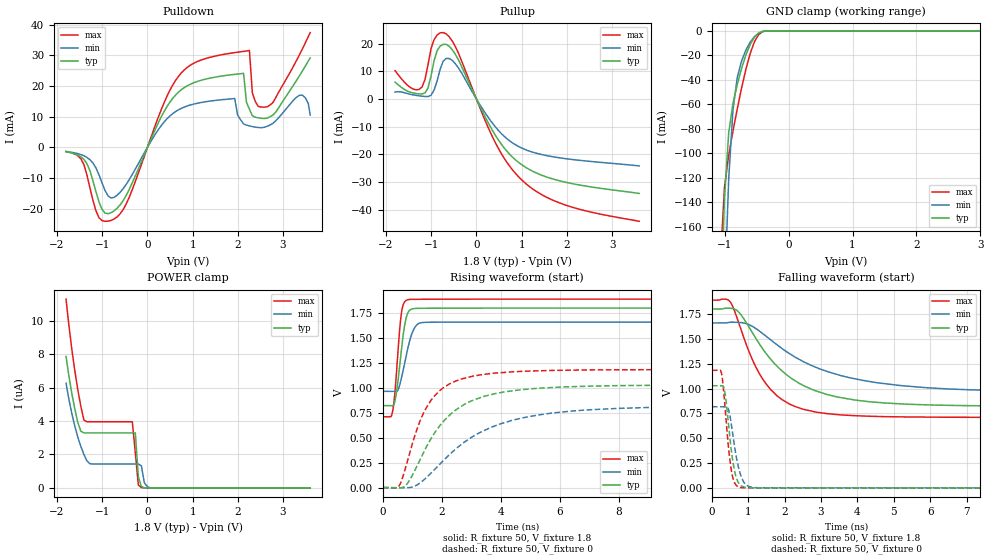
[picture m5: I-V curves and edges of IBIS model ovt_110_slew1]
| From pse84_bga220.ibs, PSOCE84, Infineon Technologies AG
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[Model] ovt_110_slew1
Model_type I/O
Enable   Active-High
Vinl  =  0.54
Vinh  =  1.26
Vmeas =  0.9
Cref  =  15e-12
| Capacitance   typ   min   max
C_comp   1.39974e-12   1.35992e-12   1.44753e-12
| Variables   typ   min   max
[GND Clamp Reference]   0   0   0
[POWER Clamp Reference]   1.8   1.66   1.89
[Pulldown Reference]   0   0   0
[Pullup Reference]   1.8   1.66   1.89
[Temperature Range]   25   125   -40
[Voltage Range]   1.8   1.66   1.89
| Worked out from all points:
|   slope of the pulldown table from 0 to 0.27 V, typ, clamps not added: 30.3 ohm
|   slope of the pullup table from 0 to 0.27 V, typ, clamps not added: 30.5 ohm
|   GND clamp passes 1 mA (typ) near -0.43 V on its own axis
|   falling waveform, R_fixture 50, V_fixture 1.8: 20-80 % time 1.54ns typ, 2.34ns min, 992ps max; typ from 1.8 V to 0.822 V
|   falling waveform, R_fixture 50, V_fixture 0: 20-80 % time 200ps typ, 233ps min, 180ps max; typ from 1.03 V to 0 V
|   rising waveform, R_fixture 50, V_fixture 1.8: 20-80 % time 234ps typ, 323ps min, 184ps max; typ from 0.822 V to 1.8 V
|   rising waveform, R_fixture 50, V_fixture 0: 20-80 % time 1.56ns typ, 2.46ns min, 1.04ns max; typ from 0 V to 1.03 V
[GND Clamp]
| Voltage   I(typ)   I(min)   I(max)
-1.271V   -717.5mA   -832.8mA   -643.6mA
-1.07V    -241.9mA   -348.3mA   -192.2mA
-1.003V   -137.2mA   -218.1mA   -128.1mA
-936.6mV  -83.06mA   -120.7mA   -101.3mA
-869.7mV  -59.26mA   -64.32mA   -81.77mA
-802.8mV  -43.7mA    -38.08mA   -63.69mA
-735.9mV  -30.76mA   -24.63mA   -46.83mA
-602.1mV  -11.27mA   -9.362mA   -18.72mA
-535.2mV  -5.241mA   -4.803mA   -9.042mA
-468.3mV  -1.746mA   -1.965mA   -3.086mA
-334.5mV  -35.9uA    -120.8uA   -33.39uA
3.6V      0A         0A         0A
[POWER Clamp]
| Voltage   I(typ)   I(min)   I(max)
-1.8V     7.872uA    6.273uA    11.31uA
-1.672V   5.671uA    4.461uA    8.32uA
-1.539V   3.91uA     3.037uA    5.87uA
-1.405V   3.295uA    2.008uA    4.063uA
-1.271V   3.295uA    1.447uA    3.964uA
-334.5mV  3.295uA    1.429uA    3.964uA
-267.6mV  3.295uA    1.429uA    2.099uA
-200.7mV  664.1nA    1.429uA    166.6nA
-133.8mV  69.92nA    1.319uA    14.86nA
-66.9mV   7.33nA     291.5nA    4.066nA
62.07mV   0A         0A         0A
3.6V      0A         0A         0A
[Pulldown]
| Voltage   I(typ)   I(min)   I(max)
-1.8V     -1.439mA   -1.35mA    -1.318mA
-1.405V   -3.905mA   -2.719mA   -5.569mA
-1.07V    -17.75mA   -8.962mA   -22.94mA
-735.9mV  -20.66mA   -16.27mA   -23.33mA
806.9mV   19.41mA    13.09mA    25.15mA
1.93V     23.81mA    15.95mA    30.9mA
2.126V    24.14mA    7.657mA    31.3mA
2.256V    12.46mA    7.006mA    31.58mA
2.321V    10.32mA    6.784mA    17.72mA
2.647V    9.522mA    6.888mA    13.22mA
3.364V    23.4mA     17mA       30.24mA
3.6V      29.19mA    10.55mA    37.43mA
[Pullup]
| Voltage   I(typ)   I(min)   I(max)
-1.8V     6.105mA    2.518mA    10.28mA
-1.271V   1.855mA    1.166mA    3.446mA
-1.137V   2.224mA    912.4uA    7.05mA
-1.07V    4.038mA    883.8uA    12.45mA
-936.6mV  13.89mA    3.25mA     21.49mA
-802.8mV  19.14mA    10.79mA    23.94mA
-669mV    19.74mA    14.67mA    23.55mA
-401.4mV  14.31mA    11.31mA    16.73mA
434.5mV   -13.51mA   -10.38mA   -16.28mA
993.1mV   -23.65mA   -17.65mA   -29.11mA
1.89V     -29.77mA   -21.37mA   -37.87mA
3.6V      -34.13mA   -24.18mA   -44.2mA
[Ramp]
dV/dt_r   0.617231/1.56317n  0.490169/2.45731n  0.709901/1.03544n
dV/dt_f   0.586718/1.54262n  0.416735/2.33681n  0.708163/0.991622n
R_load = 50
[Falling Waveform]
R_fixture = 50
V_fixture = 1.8
V_fixture_min = 1.66
V_fixture_max = 1.89
| Time   V(typ)   V(min)   V(max)
0s        1.8V       1.66V      1.89V
515.3ps   1.808V     1.668V     1.867V
775.6ps   1.754V     1.665V     1.621V
1.309ns   1.447V     1.578V     1.148V
1.615ns   1.296V     1.49V      989.8mV
2.13ns    1.117V     1.353V     844.4mV
2.82ns    980.9mV    1.219V     766.2mV
3.932ns   884.1mV    1.098V     726.6mV
6.977ns   827.7mV    988.9mV    710.3mV
800ns     822.1mV    965.4mV    709.7mV
[Falling Waveform]
R_fixture = 50
V_fixture = 0
V_fixture_min = 0
V_fixture_max = 0
| Time   V(typ)   V(min)   V(max)
0s        1.029V     816.9mV    1.183V
265.6ps   1.029V     816.9mV    1.152V
349.3ps   979.8mV    816.8mV    864.6mV
444.9ps   677.9mV    800.6mV    449.4mV
541.3ps   356.8mV    624.1mV    162.3mV
650.1ps   128.8mV    355.3mV    34.74mV
874.5ps   9.514mV    59.64mV    592.5uV
1.226ns   617.4uV    1.815mV    599.9uV
3.775ns   116.3uV    161.5uV    79.53uV
800ns     18.65nV    979.8nV    8.521nV
[Rising Waveform]
R_fixture = 50
V_fixture = 1.8
V_fixture_min = 1.66
V_fixture_max = 1.89
| Time   V(typ)   V(min)   V(max)
0s        822.1mV    965.4mV    709.7mV
267.7ps   822.4mV    965.4mV    710.1mV
335.4ps   821mV      965.6mV    770.4mV
466.2ps   962.6mV    964.4mV    1.164V
596.8ps   1.289V     1.056V     1.67V
690.7ps   1.533V     1.179V     1.834V
822.7ps   1.734V     1.365V     1.883V
1.036ns   1.794V     1.58V      1.888V
1.422ns   1.799V     1.657V     1.889V
800ns     1.8V       1.66V      1.89V
[Rising Waveform]
R_fixture = 50
V_fixture = 0
V_fixture_min = 0
V_fixture_max = 0
| Time   V(typ)   V(min)   V(max)
0s        18.66nV    979.6nV    8.526nV
558.9ps   -2.512mV   -1.689mV   19.77mV
860ps     52.43mV    -930.9uV   292.7mV
1.379ns   351.5mV    74.18mV    747.4mV
1.731ns   536.9mV    173.9mV    912.3mV
2.272ns   728.5mV    334.5mV    1.042V
2.995ns   868.1mV    501.3mV    1.113V
4.393ns   970mV      675mV      1.161V
8.356ns   1.024V     797.5mV    1.182V
800ns     1.029V     816.9mV    1.183V
